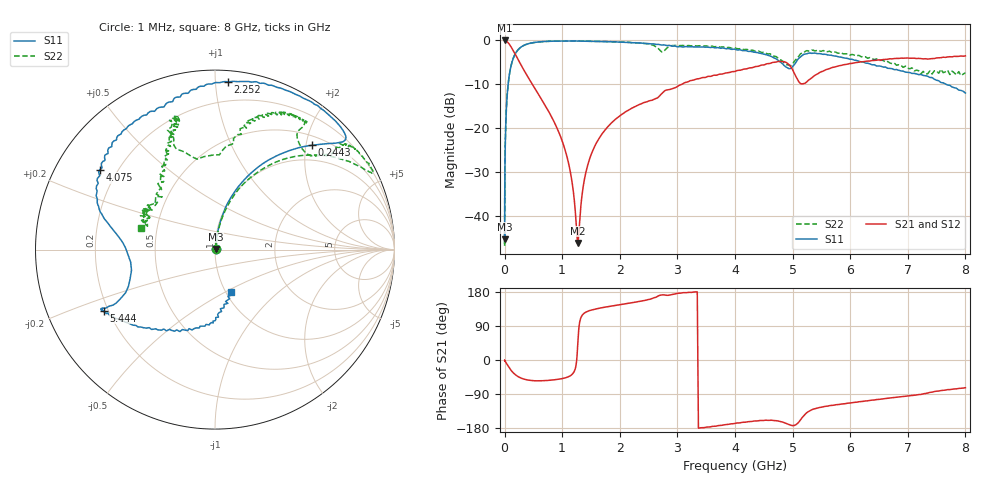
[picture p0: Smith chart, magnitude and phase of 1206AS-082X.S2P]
!s-Parameter Generated by FASTRON Sdn. Bhd.
!FASTRON P/N : 1206AS-082X
!Keysight Technologies: E5071C_MY46733604_B.14.02
!Date: Wed Nov 15 10:27:00 2023
!Version  :Rev00  Wed Nov 15 10:27:00 2023
!Data & Calibration Information:
!Freq  S11:SOLT2(ON)  S21:SOLT2(ON)  S12:SOLT2(ON)  S22:SOLT2(ON)
!PortZ  Port1:50+j0  Port2:50+j0
!When reading reference impedance value at option line is always used.
! Remarks : This data is being provided solely for informational purposes.
# Hz S dB R 50
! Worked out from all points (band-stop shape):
!   1601 points, 1 MHz to 8 GHz, reference 50 ohm
!   highest |S21| = -0.02 dB at 1.284 MHz (marker M1); lowest = -46.2 dB at 1.272 GHz (marker M2)
!   |S21| within 3 dB of the highest: start of sweep to 180.6 MHz
!   lowest |S11| = -45.3 dB at 1.053 MHz (marker M3), VSWR 1.01, Z = 50.4 + j0.331 ohm
!   |S11| at or under -10 dB: start of sweep to 62.43 MHz; 7.664 GHz to end of sweep
!   |S22| runs from -46.9 to -0.1 dB; largest |S21 - S12| = 0.0073
!   S11 on the Smith chart (normalised r, x): 1 MHz: 1.01, +0.01; 244.3 MHz: 0.67, +2.12; 2.252 GHz: 0.07, +1.08; 4.075 GHz: 0.13, +0.31; 5.444 GHz: 0.18, -0.25; 8 GHz: 1.05, -0.53
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1000000  -44.27 30.5  -0.04 -0.4  -0.05 -0.4  -45.53 38.5
1052806  -45.30 37.1  -0.04 -0.4  -0.05 -0.4  -45.59 34.1
1283835  -42.68 40.2  -0.02 -0.5  -0.06 -0.5  -44.10 51.4
4479405  -31.92 77.4  -0.05 -1.3  -0.05 -1.3  -32.01 78.9
2.00676e7  -19.28 80.9  -0.11 -5.6  -0.13 -5.5  -19.22 80.2
8.994653e7  -7.29 66.8  -1.02 -22.6  -1.02 -22.6  -7.31 64.7
2.443405e8  -2.01 47.1  -4.59 -44.6  -4.60 -44.6  -2.00 41.5
4.006501e8  -0.81 40.9  -8.23 -52.7  -8.23 -52.7  -0.82 31.6
9.292726e8  -0.16 47.0  -20.54 -50.9  -20.55 -50.9  -0.17 26.1
1.108954e9  -0.14 51.9  -27.86 -44.1  -27.87 -44.2  -0.16 27.1
1.272209e9  -0.15 56.2  -46.17 44.6  -46.23 44.6  -0.14 28.5
1.465558e9  -0.22 62.2  -27.46 129.9  -27.47 129.8  -0.21 30.2
1.7949e9  -0.32 72.0  -19.64 140.7  -19.66 140.5  -0.29 33.6
2.252141e9  -0.56 85.7  -15.18 152.1  -15.20 151.9  -0.51 38.1
2.648292e9  -0.92 97.1  -13.16 167.3  -13.20 167.1  -1.62 39.7
3.26428e9  -1.47 119.7  -9.11 178.7  -9.13 178.7  -1.22 57.0
4.075033e9  -2.14 145.3  -6.82 -166.1  -6.82 -166.1  -1.92 68.1
4.772513e9  -4.82 169.3  -4.79 -161.8  -4.76 -162.0  -4.38 80.0
5.080423e9  -4.53 -152.6  -8.78 -168.2  -8.76 -168.4  -4.08 111.5
5.444317e9  -3.04 -151.1  -7.56 -126.0  -7.53 -126.3  -2.22 106.7
6.72769e9  -6.45 -108.6  -4.22 -99.6  -4.19 -100.1  -5.29 119.4
8e9  -12.00 -69.6  -3.54 -73.1  -3.52 -73.6  -7.38 163.7
